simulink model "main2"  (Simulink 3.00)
settings: Solver=ode45  StartTime=0.0  StopTime=9999999  RelTol=1e-3

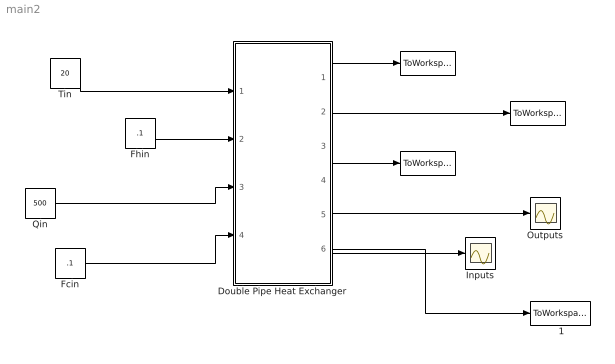
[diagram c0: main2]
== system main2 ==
  " " : ToWorkspace  VariableName=Thout  SampleTime=-1  SaveFormat=Matrix
  "  " : ToWorkspace  VariableName=Thin  SampleTime=-1  SaveFormat=Matrix
  "   " : ToWorkspace  VariableName=Thm  SampleTime=-1  SaveFormat=Matrix
  " 1" : ToWorkspace  VariableName=Tcout  SampleTime=-1  SaveFormat=Matrix
  Double Pipe Heat Exchanger : Subsystem  mask{tstep=.1, Cpw=1.0, rhow=1.0, Cpheat=0.1, Mheat=27.3, Uheat=0.9, Upipe=1.8, oDodpipe=0.5, iDodpipe=0.43, oDidpipe=0.375, iDidpipe=0.31, Lpipe=35.0, oDhpipe=0.5, iDhpipe=0.43, Dheat=0.375, Lheat=2.5}
      mask prompts: tstep "Simulation time step (sec):"; Cpw "Specific Heat of Water (cal/g deg C)"; rhow "Density of Water (g/mL)"; Cpheat "Specific Heat of the heater (cal/g deg C)"; Mheat "Mass of Heater (g)"; Uheat "Overall Heat Transfer Coefficient for the Heater (kW/m^2 deg C)"; Upipe "Overall Heat Transfer Coefficient for the Pipe (kW/m^2 deg C)"; oDodpipe "Outer Diameter of the outer double pipe (in)"; iDodpipe "Inner diameter of the outer double pipe (in)"; oDidpipe "Outer diameter of the inner double pipe (in)"; iDidpipe "Inner diameter of the inner double pipe (in)"; Lpipe "Length of the pipe exchanger (in)"; oDhpipe "Outer diameter of the pipe surrounding the heater (in)"; iDhpipe "Inner diameter of the pipe surrounding the heater (in)"; Dheat "Diameter of the heater (in)"; Lheat "Length of the heater (in)"
      mask init:
      | Param(1)=tstep;
      | Param(2)=Cpw;
      | Param(3)=rhow;
      | Param(4)=Cpheat;
      | Param(5)=Mheat;
      | Param(7)=Uheat;
      | Param(8)=Upipe;
      | Param(9)=oDodpipe;
      | Param(10)=iDodpipe;
      | Param(11)=oDidpipe;
      | Param(12)=iDidpipe;
      | Param(13)=Lpipe;
      | Param(14)=oDhpipe;
      | Param(15)=iDhpipe;
      | Param(16)=Dheat;
      | Param(17)=Lheat;
      | rhoheat=Mheat/((pi*(Dheat/2)^2*Lheat)*2.54^3);
      | Param(6)=rhoheat;
  Fcin : Constant  Value=.1
  Fhin : Constant  Value=.1
  Inputs : Scope
  Outputs : Scope
  Qin : Constant  Value=500
  Tin : Constant  Value=20
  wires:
  Double Pipe Heat Exchanger/1(Thin) -> "  "/1
  Double Pipe Heat Exchanger/2(Thm) -> "   "/1
  Double Pipe Heat Exchanger/4(Outputs) -> Outputs/1
  Tin/1 -> Double Pipe Heat Exchanger/1(Tin)
  Double Pipe Heat Exchanger/5(Inputs) -> Inputs/1
  Fhin/1 -> Double Pipe Heat Exchanger/2(Fhin)
  Double Pipe Heat Exchanger/3(Thout) -> " "/1
  Double Pipe Heat Exchanger/6(Tcout) -> " 1"/1
  Qin/1 -> Double Pipe Heat Exchanger/3(Qin)
  Fcin/1 -> Double Pipe Heat Exchanger/4(Fcin)

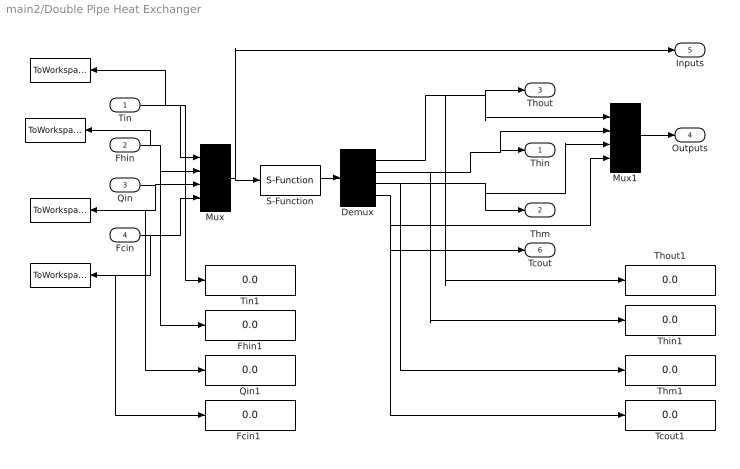
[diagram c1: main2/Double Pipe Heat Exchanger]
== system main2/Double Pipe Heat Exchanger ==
  Tin : Inport  Port=1  PortWidth=-1  SampleTime=-1  DataType=auto
  Fhin : Inport  Port=2  PortWidth=-1  SampleTime=-1  DataType=auto
  Qin : Inport  Port=3  PortWidth=-1  SampleTime=-1  DataType=auto
  Fcin : Inport  Port=4  PortWidth=-1  SampleTime=-1  DataType=auto
  "  " : ToWorkspace  VariableName=Tin  SampleTime=-1  SaveFormat=Matrix
  "   " : ToWorkspace  VariableName=Fhin  SampleTime=-1  SaveFormat=Matrix
  "     " : ToWorkspace  VariableName=Qin  SampleTime=-1  SaveFormat=Matrix
  "      " : ToWorkspace  VariableName=Fcin  SampleTime=-1  SaveFormat=Matrix
  Demux : Demux  Outputs=4
  "Fcin1 " : Display
  Fhin1 : Display
  Mux : Mux  Inputs=4
  Mux1 : Mux  Inputs=4
  Qin1 : Display
  S-Function : S-Function  FunctionName=heatx  Parameters=Param  PortCounts=[]  SFunctionModules=''
  Tcout1 : Display
  Thin1 : Display
  Thm1 : Display
  Thout1 : Display
  Tin1 : Display
  Thin : Outport  Port=1
  Thm : Outport  Port=2
  Thout : Outport  Port=3
  Outputs : Outport  Port=4
  Inputs : Outport  Port=5
  Tcout : Outport  Port=6
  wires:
  S-Function/1 -> Demux/1
  Mux1/1 -> Outputs/1
  Mux/1 -> S-Function/1, Inputs/1
  Tin/1 -> Mux/1, "  "/1, Tin1/1
  Fhin/1 -> "   "/1, Mux/2, Fhin1/1
  Fcin/1 -> Mux/4, "      "/1, "Fcin1 "/1
  Qin/1 -> Mux/3, "     "/1, Qin1/1
  Demux/4 -> Mux1/4, Tcout/1, Tcout1/1
  Demux/1 -> Thout/1, Mux1/1, Thout1/1
  Demux/2 -> Thin/1, Mux1/2, Thin1/1
  Demux/3 -> Thm/1, Mux1/3, Thm1/1
